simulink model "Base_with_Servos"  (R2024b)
settings: Solver=VariableStepAuto  StartTime=0.0  StopTime=10.0  RelTol=1e-3
undefined symbols (not defined in the file): kg, m, s, X, Y, Z
libraries: sm_lib x7, nesl_utility x1

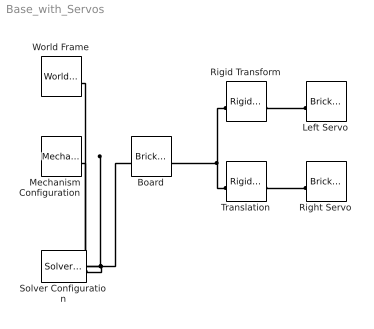
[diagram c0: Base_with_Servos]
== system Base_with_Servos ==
  Board : sm_lib/Body Elements/Brick Solid  BrickDimensions=[30 30 4]  BrickDimensionsUnits=cm  ExportEntireGeometry=off  InertiaType=CalculateFromGeometry  BasedOnType=Density  Density=1000  DensityUnits=kg/m^3  Mass=1  MassUnits=kg  CenterOfMass=[0 0 0]  CenterOfMassUnits=m  MomentsOfInertia=[1 1 1]  MomentsOfInertiaUnits=kg*m^2  ProductsOfInertia=[0 0 0]  ProductsOfInertiaUnits=kg*m^2  GraphicType=FromGeometry  MarkerShape=Sphere  MarkerSize=10  GraphicVisPropType=SimpleVisualProperties  GraphicDiffuseColor=[1 1 0.06667]  GraphicOpacity=1  GraphicSpecularColor=[0.5 0.5 0.5 1.0]  GraphicAmbientColor=[0.15 0.15 0.15 1.0]  GraphicEmissiveColor=[0.0 0.0 0.0 1.0]  GraphicShininess=75  DoExposeReferenceFrame=on  SerializedFrames=<Frames><Frame><Id>Frame1</Id><Value><Name>F1</Name><Origin><Source>ReferenceFrame</Source><FeatureName></FeatureName></Origin><PrimaryAxis><DefinedDirection>+Z</DefinedDirection><Source>ReferenceFrame</Source><SourceDirection>+Z</SourceDirection><FeatureName></FeatureName></PrimaryAxis><SecondaryAxis><DefinedDirection>+X</DefinedDirection><Source>ReferenceFrame</Source><SourceDirection>+X</Source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
  Left Servo : sm_lib/Body Elements/Brick Solid  BrickDimensions=[5.7 2.7 5]  BrickDimensionsUnits=cm  ExportEntireGeometry=off  InertiaType=CalculateFromGeometry  BasedOnType=Density  Density=1000  DensityUnits=kg/m^3  Mass=1  MassUnits=kg  CenterOfMass=[0 0 0]  CenterOfMassUnits=m  MomentsOfInertia=[1 1 1]  MomentsOfInertiaUnits=kg*m^2  ProductsOfInertia=[0 0 0]  ProductsOfInertiaUnits=kg*m^2  GraphicType=FromGeometry  MarkerShape=Sphere  MarkerSize=10  GraphicVisPropType=SimpleVisualProperties  GraphicDiffuseColor=[0.5 0.5 0.5]  GraphicOpacity=1  GraphicSpecularColor=[0.5 0.5 0.5 1.0]  GraphicAmbientColor=[0.15 0.15 0.15 1.0]  GraphicEmissiveColor=[0.0 0.0 0.0 1.0]  GraphicShininess=75  DoExposeReferenceFrame=on  SerializedFrames=<Frames><Frame><Id>Frame1</Id><Value><Name>F1</Name><Origin><Source>ReferenceFrame</Source><FeatureName></FeatureName></Origin><PrimaryAxis><DefinedDirection>+Z</DefinedDirection><Source>ReferenceFrame</Source><SourceDirection>+Z</SourceDirection><FeatureName></FeatureName></PrimaryAxis><SecondaryAxis><DefinedDirection>+X</DefinedDirection><Source>ReferenceFrame</Source><SourceDirection>+X</Source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
  Mechanism Configuration : sm_lib/Utilities/Mechanism Configuration  UniformGravity=Constant  GravityVector=[0 0 -9.80665]  GravityVectorUnits=m/s^2  LinearizationDelta=0.001  JointModeTransitionNonlinearIterations=2
  Right Servo : sm_lib/Body Elements/Brick Solid  BrickDimensions=[5.7 2.7 5]  BrickDimensionsUnits=cm  ExportEntireGeometry=off  InertiaType=CalculateFromGeometry  BasedOnType=Density  Density=1000  DensityUnits=kg/m^3  Mass=1  MassUnits=kg  CenterOfMass=[0 0 0]  CenterOfMassUnits=m  MomentsOfInertia=[1 1 1]  MomentsOfInertiaUnits=kg*m^2  ProductsOfInertia=[0 0 0]  ProductsOfInertiaUnits=kg*m^2  GraphicType=FromGeometry  MarkerShape=Sphere  MarkerSize=10  GraphicVisPropType=SimpleVisualProperties  GraphicDiffuseColor=[0.5 0.5 0.5]  GraphicOpacity=1  GraphicSpecularColor=[0.5 0.5 0.5 1.0]  GraphicAmbientColor=[0.15 0.15 0.15 1.0]  GraphicEmissiveColor=[0.0 0.0 0.0 1.0]  GraphicShininess=75  DoExposeReferenceFrame=on  SerializedFrames=<Frames><Frame><Id>Frame1</Id><Value><Name>F1</Name><Origin><Source>ReferenceFrame</Source><FeatureName></FeatureName></Origin><PrimaryAxis><DefinedDirection>+Z</DefinedDirection><Source>ReferenceFrame</Source><SourceDirection>+Z</SourceDirection><FeatureName></FeatureName></PrimaryAxis><SecondaryAxis><DefinedDirection>+X</DefinedDirection><Source>ReferenceFrame</Source><SourceDirection>+X</Source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
  Rigid Transform : sm_lib/Frames and Transforms/Rigid Transform  RotationMethod=None  FollAlignAxisA=+X  BaseAlignAxisA=+Y  FollAlignAxisB=+Y  BaseAlignAxisB=+Z  RotationStandardAxis=+Z  RotationAngle=0  RotationAngleUnits=deg  RotationArbitraryAxis=[0 0 1]  RotationSequenceAxes=FollowerAxes  RotationSequence=XYX  RotationSequenceAngles=[0 0 0]  RotationSequenceAnglesUnits=deg  RotationMatrix=[1 0 0;0 1 0;0 0 1]  Quaternion=[1 0 0 0]  TranslationMethod=Cartesian  TranslationCartesianOffset=[-3.8 -16.8 0.5]  TranslationCartesianOffsetUnits=cm  TranslationStandardAxis=+Z  TranslationStandardOffset=0  TranslationStandardOffsetUnits=m  TranslationROffset=0  TranslationROffsetUnits=m  TranslationThetaOffset=0  TranslationThetaOffsetUnits=deg  TranslationZOffset=0  TranslationZOffsetUnits=m
  Solver Configuration : nesl_utility/Solver Configuration  PhysicalDomain=network_engine_domain  SubClassName=solver  LeftPortType=input  RightPortType=generic  Tones=[]  Harmonics=[]  SimulateNoise=off  Profile=off  UseLocalSampling=off  EnableSwitchedLinearOptims=on  FrequencyDomain=off  UseCCode=off  RelTol=0.001  AbsTol=0.001  MinStep=1e-09  ToWorkspace=off  RevertToSquareIcSolve=off  NumHomotopyIterations=100  PhasorMode=off  PhasorModeNumHarmonics=1  ConsistencySolver=NEWTON_XTOL_AFTER_FTOL  IndexReductionMethod=DerivativeReplacement  DoDC=off  ResidualTolerance=1e-09  ConsistencyTolSource=GLOBAL  ConsistencyAbsTol=0.001  ConsistencyRelTol=0.001  ConsistencyTolFactor=0.001  UseLocalSolver=off  LocalSolverChoice=NE_BACKWARD_EULER_ADVANCER  ResolveIndetEquations=on  FunctionEvalNumThread=1  LocalSolverSampleTime=0.001  DoFixedCost=off  MaxNonlinIter=3  MaxModeIter=2  ComputeImpulses=off  ImpulseIterations=2  LinearAlgebra=auto  LinearAlgebraNumThread=0  EquationFormulation=NE_TIME_EF  DelaysMemoryBudget=1024  AutomaticFiltering=on  FilteringTimeConstant=0.001  PartitionStorageMethod=AS_NEEDED  PartitionMemoryBudget=1024  PartitionMethod=ROBUST  MultibodyUseLocalSolver=off  MultibodyLocalSolverChoice=ODE1  MultibodyLocalSolverSampleTime=0.001
  Translation : sm_lib/Frames and Transforms/Rigid Transform  RotationMethod=StandardAxis  FollAlignAxisA=+X  BaseAlignAxisA=+Y  FollAlignAxisB=+Y  BaseAlignAxisB=+Z  RotationStandardAxis=+Z  RotationAngle=180  RotationAngleUnits=deg  RotationArbitraryAxis=[0 0 1]  RotationSequenceAxes=FollowerAxes  RotationSequence=XYX  RotationSequenceAngles=[0 0 0]  RotationSequenceAnglesUnits=deg  RotationMatrix=[1 0 0;0 1 0;0 0 1]  Quaternion=[1 0 0 0]  TranslationMethod=Cartesian  TranslationCartesianOffset=[3.8 -16.8 0.5]  TranslationCartesianOffsetUnits=cm  TranslationStandardAxis=+Z  TranslationStandardOffset=0  TranslationStandardOffsetUnits=m  TranslationROffset=0  TranslationROffsetUnits=m  TranslationThetaOffset=0  TranslationThetaOffsetUnits=deg  TranslationZOffset=0  TranslationZOffsetUnits=m
  World Frame : sm_lib/Frames and Transforms/World Frame
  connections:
  Solver Configuration/RConn1 -- Mechanism Configuration/RConn1 -- Board/LConn1 -- World Frame/RConn1
  Translation/LConn1 -- Board/RConn1 -- Rigid Transform/LConn1
  Rigid Transform/RConn1 -- Left Servo/LConn1
  Right Servo/LConn1 -- Translation/RConn1
